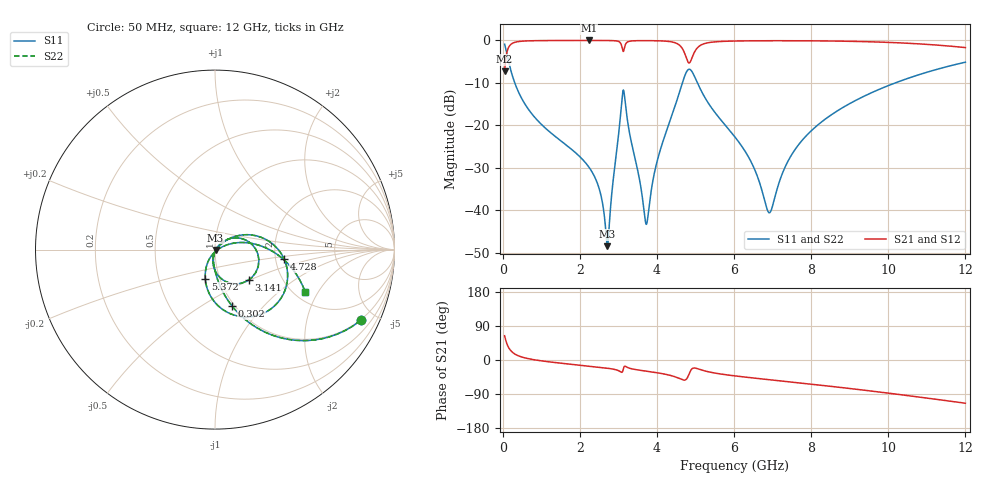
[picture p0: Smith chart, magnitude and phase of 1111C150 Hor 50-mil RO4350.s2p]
# GHz S MA R 50
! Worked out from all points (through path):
!   11951 points, 50 MHz to 12 GHz, reference 50 ohm
!   highest |S21| = -0.02 dB at 2.241 GHz (marker M1); lowest = -7.3 dB at 50 MHz (marker M2)
!   group delay of S21, straight-line fit = 27.3 ps
!   lowest |S11| = -48.4 dB at 2.717 GHz (marker M3), VSWR 1.01, Z = 50.3 - j0.183 ohm
!   |S11| at or under -10 dB: 313.5 MHz to 4.661 GHz (4.348 GHz wide, 175 % of centre); 5.051 GHz to 10.18 GHz (5.134 GHz wide, 67.4 % of centre)
!   |S22| runs from -48.4 to -0.9 dB; largest |S21 - S12| = 0
!   S11 on the Smith chart (normalised r, x): 50 MHz: 0.97, -4.12; 302 MHz: 0.97, -0.68; 3.141 GHz: 1.36, -0.49; 4.728 GHz: 2.23, -0.27; 5.372 GHz: 0.85, -0.29; 12 GHz: 2.29, -1.54
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0.05  0.9021 -26.0  0.4315 64.0  0.4315 64.0  0.9021 -26.0
0.173  0.517 -60.2  0.8556 29.7  0.8556 29.7  0.517 -60.2
0.302  0.327 -73.3  0.9445 16.6  0.9445 16.6  0.327 -73.3
0.838  0.1233 -89.3  0.9915 0.3  0.9915 0.3  0.1233 -89.3
2.042  0.041 -102.0  0.9975 -14.1  0.9975 -14.1  0.041 -102.0
2.241  0.03202 -103.1  0.9976 -16.2  0.9976 -16.2  0.03202 -103.1
2.516  0.01713 -101.2  0.9973 -19.2  0.9973 -19.2  0.01713 -101.2
2.717  0.003788 -28.7  0.9961 -21.7  0.9961 -21.7  0.003788 -28.7
3.04  0.1108 34.6  0.9473 -30.0  0.9473 -30.0  0.1108 34.6
3.141  0.2532 -41.9  0.7611 -19.5  0.7611 -19.5  0.2532 -41.9
3.263  0.09527 -94.4  0.9689 -20.7  0.9689 -20.7  0.09527 -94.4
3.713  0.00699 -42.9  0.993 -29.3  0.993 -29.3  0.00699 -42.9
4.034  0.04231 41.3  0.9883 -34.2  0.9883 -34.2  0.04231 41.3
4.728  0.3882 -7.7  0.6876 -52.9  0.6876 -52.9  0.3882 -7.7
4.926  0.4167 -64.2  0.6504 -22.2  0.6504 -22.2  0.4167 -64.2
5.372  0.1718 -108.3  0.9453 -31.9  0.9453 -31.9  0.1718 -108.3
6.025  0.07276 -120.3  0.9824 -42.0  0.9824 -42.0  0.07276 -120.3
6.917  0.009358 -49.2  0.9903 -52.0  0.9903 -52.0  0.009358 -49.2
7.397  0.03773 19.8  0.9905 -57.2  0.9905 -57.2  0.03773 19.8
8.017  0.08754 20.8  0.9877 -64.0  0.9877 -64.0  0.08754 20.8
10.009  0.2946 0.8  0.9467 -87.5  0.9467 -87.5  0.2946 0.8
12  0.5536 -25.0  0.8228 -114.0  0.8228 -114.0  0.5536 -25.0
